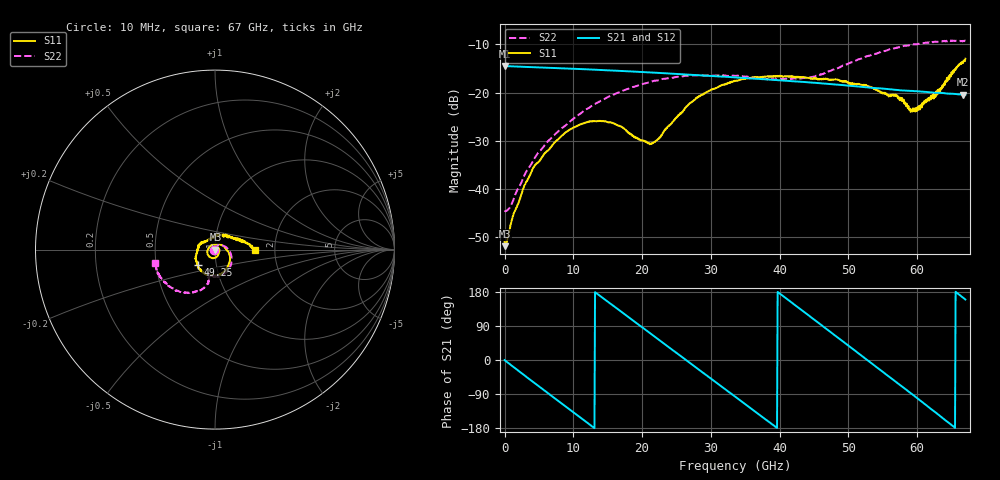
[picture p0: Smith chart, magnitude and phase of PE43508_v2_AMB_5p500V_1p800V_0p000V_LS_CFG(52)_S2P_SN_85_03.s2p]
!Keysight Technologies,N5227A,US51270237,A.10.43.00
!Date: Wednesday, August 22, 2018 17:12:01
!Correction: S11(Full 2 Port(1,3))
!S31(Full 2 Port(1,3))
!S13(Full 2 Port(1,3))
!S33(Full 2 Port(1,3))
!S2P File: Measurements: S11, S31, S13, S33:
# Hz S  dB  R 50
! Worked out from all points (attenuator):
!   801 points, 10 MHz to 67 GHz, reference 50 ohm
!   highest |S21| = -14.49 dB at 10 MHz (marker M1); lowest = -20.5 dB at 66.67 GHz (marker M2)
!   lowest |S11| = -51.9 dB at 93.74 MHz (marker M3), VSWR 1.01, Z = 50.3 + j0.01 ohm
!   |S11| at or under -10 dB: start of sweep to end of sweep
!   |S22| runs from -44.8 to -9.2 dB; largest |S21 - S12| = 0.00098
!   S11 on the Smith chart (normalised r, x): 10 MHz: 1.01, -0.00; 49.25 GHz: 0.81, -0.14; 67 GHz: 1.58, -0.01
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1e7  -51.03 -9.2  -14.49 -0.2  -14.50 -0.2  -44.76 -178.3
9.37375e7  -51.90 2.2  -14.51 -1.4  -14.52 -1.5  -44.64 174.5
9.311125e8  -47.20 17.4  -14.57 -13.3  -14.57 -13.3  -43.51 132.0
2.773338e9  -39.86 5.1  -14.67 -39.0  -14.67 -39.0  -37.57 86.5
4.280612e9  -35.38 -11.6  -14.75 -59.8  -14.75 -59.7  -33.88 67.5
8.467488e9  -28.78 -63.5  -14.98 -117.1  -14.97 -117.1  -27.26 34.5
1.123082e10  -26.49 -94.2  -15.14 -154.8  -15.15 -154.8  -24.15 12.6
1.449659e10  -25.95 -132.9  -15.35 160.8  -15.35 160.8  -21.36 -10.0
1.759488e10  -27.73 -175.5  -15.57 118.8  -15.57 118.8  -19.43 -29.2
2.102811e10  -30.52 105.0  -15.83 72.3  -15.82 72.3  -17.92 -49.1
2.236791e10  -29.67 64.9  -15.93 54.2  -15.92 54.2  -17.43 -56.2
2.789459e10  -21.21 -21.0  -16.37 -20.6  -16.38 -20.6  -16.43 -81.3
3.3505e10  -17.60 -66.8  -16.86 -96.4  -16.87 -96.4  -16.53 -99.7
3.911541e10  -16.71 -98.7  -17.37 -172.5  -17.38 -172.4  -17.32 -106.3
4.472582e10  -17.10 -122.5  -17.94 110.6  -17.93 110.6  -16.77 -103.1
4.924765e10  -17.76 -138.5  -18.47 48.2  -18.48 48.2  -14.44 -101.7
5.586291e10  -20.82 174.2  -19.28 -43.5  -19.28 -43.8  -11.09 -120.4
5.912868e10  -23.54 129.2  -19.66 -88.5  -19.67 -88.7  -10.08 -133.2
6.004979e10  -22.99 103.6  -19.74 -101.5  -19.75 -101.8  -9.97 -137.1
6.29806e10  -19.44 48.3  -20.03 -142.9  -20.06 -143.2  -9.48 -149.7
6.666505e10  -13.86 3.3  -20.45 164.4  -20.53 164.5  -9.27 -165.6
6.7e10  -12.99 -0.4  -20.45 159.5  -20.52 159.6  -9.28 -167.8
